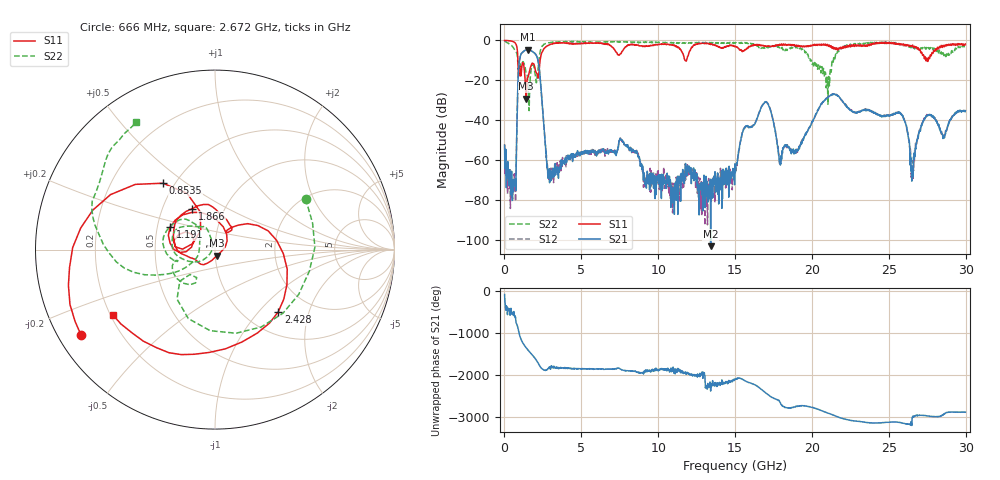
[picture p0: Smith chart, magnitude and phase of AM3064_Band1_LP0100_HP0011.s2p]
# Hz S DB R 50.0
!freq dBS11 angS11 dBS21 angS21 dBS12 angS12 dBS22 angS22
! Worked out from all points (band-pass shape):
!   1600 points, 10 MHz to 29.98 GHz, reference 50 ohm
!   highest |S21| = -4.54 dB at 1.528 GHz (marker M1); lowest = -102.9 dB at 13.41 GHz (marker M2)
!   |S21| within 3 dB of the highest: 1.046 GHz to 2.074 GHz (1.029 GHz wide, 65.9 % of centre)
!   lowest |S11| = -29.1 dB at 1.416 GHz (marker M3), VSWR 1.07, Z = 50.9 - j3.44 ohm
!   |S11| at or under -10 dB: 876.6 MHz to 2.317 GHz (1.44 GHz wide, 90.2 % of centre); 11.75 GHz to 11.84 GHz (90.72 MHz wide, 0.769 % of centre); 27.51105 GHz to 27.5531 GHz (42.04 MHz wide, 0.153 % of centre)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
!   |S22| runs from -35.1 to -0.4 dB; largest |S21 - S12| = 0.0077
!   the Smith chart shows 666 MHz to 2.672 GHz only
!   S11 on the Smith chart (normalised r, x): 666 MHz: 0.07, -0.29; 853.5 MHz: 0.43, +0.41; 1.191 GHz: 0.58, +0.16; 1.866 GHz: 0.71, +0.35; 2.428 GHz: 1.40, -1.29; 2.672 GHz: 0.21, -0.28
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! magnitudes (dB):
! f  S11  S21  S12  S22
! 10 MHz  0.0  -52.5  -51.9  -0.4
! 666 MHz  -1.1  -72.6  -67.0  -4.8
! 853.5 MHz  -6.6  -28.1  -28.0  -9.2
! 1.191 GHz  -11.1  -5.9  -5.8  -10.6
! 1.416 GHz  -29.1  -4.7  -4.6  -16.6
! 1.528 GHz  -18.5  -4.5  -4.5  -21.7
! 1.866 GHz  -11.7  -5.8  -5.8  -12.1
! 2.428 GHz  -6.1  -29.0  -29.0  -3.1
! 2.672 GHz  -3.4  -52.7  -53.6  -1.6
! 2.972 GHz  -2.0  -64.3  -68.8  -1.1
! 5.015 GHz  -1.4  -55.9  -56.7  -0.7
! 10 GHz  -2.0  -68.3  -65.2  -0.9
! 13.41 GHz  -2.0  -102.9  -71.6  -1.3
! 15 GHz  -3.0  -64.6  -67.1  -1.4
! 16.92 GHz  -2.8  -31.0  -31.0  -3.9
! 17.95 GHz  -2.3  -62.3  -61.5  -3.3
! 19.99 GHz  -2.8  -41.2  -41.1  -11.1
! 25 GHz  -1.0  -37.6  -37.2  -1.2
! 25.95 GHz  -1.7  -38.6  -38.1  -2.7
! 26.57 GHz  -2.8  -67.0  -69.0  -4.1
! 27.43 GHz  -10.2  -38.0  -38.0  -3.9
! 29.98 GHz  -1.8  -35.1  -35.4  -2.8
